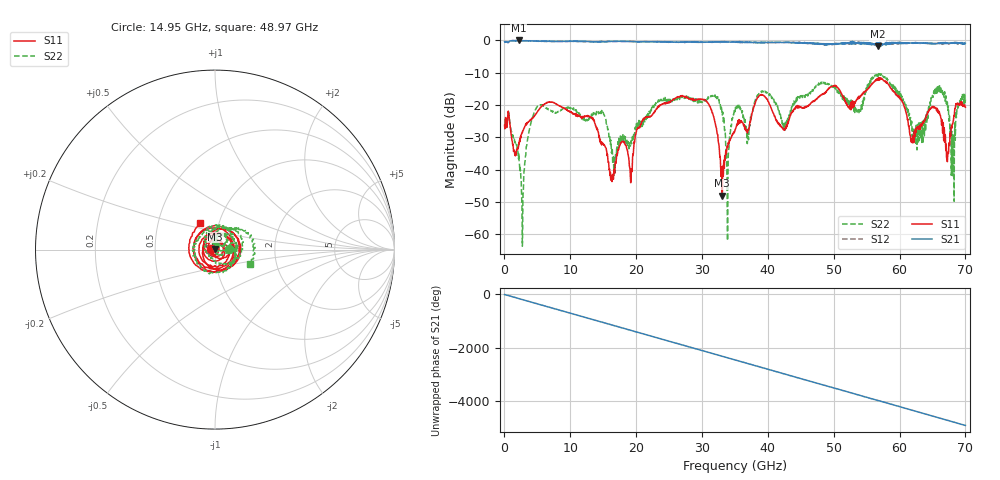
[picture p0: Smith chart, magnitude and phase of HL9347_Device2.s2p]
! 4/22/2025 2:30:34 PM
! H:\PROTOTYPE_DATA\DC_FEEDER_67GHZ\PROTO2.S2P
! CHANNEL.1
! TR.MEASUREMENT
! CORRECTED.DATA
# GHZ S RI R 50.0
! FREQ.GHZ  S11RE  S11IM  S21RE  S21IM  S12RE  S12IM  S22RE  S22IM
!; PortSelection: Port_12
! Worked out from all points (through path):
!   2000 points, 35 MHz to 70 GHz, reference 50 ohm
!   highest |S21| = -0.09 dB at 2.205 GHz (marker M1); lowest = -1.9 dB at 56.7 GHz (marker M2)
!   group delay of S21, straight-line fit = 195 ps
!   lowest |S11| = -48.1 dB at 33.08 GHz (marker M3), VSWR 1.01, Z = 50.1 + j0.383 ohm
!   |S11| at or under -10 dB: start of sweep to end of sweep
!   |S22| runs from -63.7 to -10.3 dB; largest |S21 - S12| = 0.13
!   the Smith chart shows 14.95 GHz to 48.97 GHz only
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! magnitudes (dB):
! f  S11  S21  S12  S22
! 35 MHz  -26.3  -0.5  -0.5  -26.3
! 2.205 GHz  -31.7  -0.1  -0.1  -35.0
! 2.835 GHz  -27.9  -0.2  -0.2  -47.5
! 5.215 GHz  -21.5  -0.3  -0.3  -20.2
! 11.72 GHz  -23.8  -0.4  -0.3  -23.7
! 14.95 GHz  -32.1  -0.4  -0.4  -22.2
! 16.38 GHz  -42.8  -0.4  -0.4  -33.7
! 23.38 GHz  -20.5  -0.5  -0.5  -18.5
! 30.7 GHz  -19.0  -0.6  -0.7  -18.5
! 33.08 GHz  -48.1  -0.6  -0.6  -23.2
! 33.91 GHz  -33.2  -0.6  -0.6  -55.7
! 35.03 GHz  -27.7  -0.6  -0.6  -21.9
! 42.59 GHz  -27.8  -0.7  -0.7  -27.2
! 46.69 GHz  -19.2  -1.0  -1.0  -16.0
! 53.76 GHz  -17.7  -0.9  -0.7  -21.6
! 56.7 GHz  -12.4  -1.9  -1.5  -11.0
! 58.34 GHz  -13.9  -1.1  -0.9  -12.8
! 62.3 GHz  -29.2  -1.0  -0.8  -30.6
! 66.25 GHz  -24.0  -0.8  -1.1  -14.7
! 67.23 GHz  -37.5  -1.0  -0.9  -18.5
! 68 GHz  -26.0  -0.9  -0.9  -36.6
! 70 GHz  -20.7  -1.0  -1.1  -18.4
